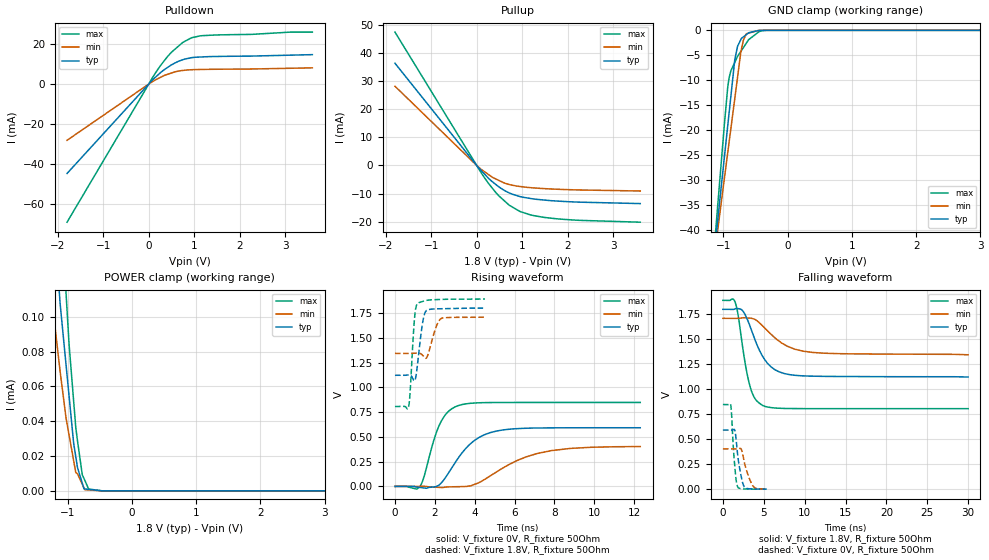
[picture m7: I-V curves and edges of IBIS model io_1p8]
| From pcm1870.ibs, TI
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|   io_1p8 Model
[Model]   io_1p8
Model_type   I/O
Polarity   Non-Inverting
Enable   Active-Low
Vinl = 0.54
Vinh = 1.26
Vmeas = 0.9
Vref = 0.9
Cref = 400pF
Rref = 50
|   typ   min   max
C_comp   2.080e-12   1.781e-12   2.321e-12
[Model spec]
Vinl   0.54   0.513   0.567
Vinh   1.26   1.197   1.323
| Where nom  PVT is Nominal Process, 1.8V, 26C
|   Fast PVT is Strong Process,  1.89V, -40C
|   Slow PVT is Weak Process,   1.71V, 86C
[Voltage Range]   1.8   1.71   1.89
|Ambient Temperature   25   85   -40
|Junction Temperature
[Temperature Range]   26   86   -40
[Pullup Reference]   1.8   1.71   1.89
[Pulldown Reference]   0   0   0
[Power Clamp Reference]   1.8   1.71   1.89
[GND Clamp Reference]   0   0   0
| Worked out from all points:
|   slope of the pulldown table from 0 to 0.27 V, typ, clamps not added: 45.5 ohm
|   slope of the pullup table from 0 to 0.27 V, typ, clamps not added: 57 ohm
|   GND clamp passes 1 mA (typ) near -0.66 V on its own axis
|   falling waveform, V_fixture 1.8V, R_fixture 50Ohm: 20-80 % time 2.31ns typ, 3.44ns min, 1.35ns max; typ from 1.8 V to 1.12 V
|   rising waveform, V_fixture 0V, R_fixture 50Ohm: 20-80 % time 1.43ns typ, 2.4ns min, 824ps max; typ from 0 V to 0.592 V
|   rising waveform, V_fixture 1.8V, R_fixture 50Ohm: 20-80 % time 253ps typ, 336ps min, 190ps max; typ from 1.12 V to 1.8 V
|   falling waveform, V_fixture 0V, R_fixture 50Ohm: 20-80 % time 615ps typ, 872ps min, 408ps max; typ from 0.592 V to 0.001 V
[Pulldown]
|   Voltage   I(typ)   I(min)   I(max)
-1.8V     -44.87mA   -28.23mA   -69.29mA
21.6mV    581uA      343.8uA    910.7uA
178.8mV   4.089mA    2.437mA    6.681mA
333mV     7.078mA    4.214mA    11.46mA
486.9mV   9.444mA    5.428mA    15.66mA
747.7mV   12.18mA    6.802mA    20.86mA
948.1mV   13.24mA    7.173mA    23.24mA
1.177V    13.59mA    7.312mA    24.25mA
2.254V    14mA       7.529mA    24.88mA
3.127V    14.48mA    7.903mA    26.04mA
3.6V      14.73mA    8.105mA    26.04mA
[GND Clamp]
|   Voltage   I(typ)   I(min)   I(max)
-1.8V     -127.5mA   -112.9mA   -149.8mA
-1.095V   -38.91mA   -40.76mA   -36.05mA
-1.053V   -33.64mA   -36.46mA   -29.45mA
-987.3mV  -25.68mA   -29.91mA   -19.15mA
-934.4mV  -19.28mA   -24.66mA   -11.54mA
-909.8mV  -16.3mA    -22.23mA   -9.421mA
-826.2mV  -6.18mA    -13.94mA   -6.495mA
-781.2mV  -3.227mA   -9.481mA   -5.246mA
-727.8mV  -1.815mA   -4.252mA   -4.205mA
-642.3mV  -852.2uA   -679uA     -2.537mA
-348.5mV  -1.381uA   0A         -19.61uA
3.6V      0A         0A         0A
[Pullup]
|   Voltage   I(typ)   I(min)   I(max)
-1.8V     36.4mA     28.23mA    47.51mA
630uV     -48.19uA   -32.61uA   -67.08uA
103.2mV   -1.872mA   -1.451mA   -2.731mA
257.4mV   -4.547mA   -3.209mA   -6.348mA
409.4mV   -6.639mA   -4.724mA   -9.437mA
563.4mV   -8.454mA   -5.933mA   -11.94mA
715.6mV   -9.781mA   -6.799mA   -14.16mA
953.7mV   -11.08mA   -7.49mA    -16.4mA
1.177V    -11.74mA   -7.897mA   -17.59mA
1.481V    -12.32mA   -8.247mA   -18.5mA
2.251V    -13.07mA   -8.732mA   -19.55mA
3.6V      -13.58mA   -9.102mA   -20.21mA
[POWER Clamp]
|   Voltage   I(typ)   I(min)   I(max)
-1.8V     770.7uA    464.9uA    734.5uA
-1.339V   212.5uA    146.7uA    327.1uA
-1.219V   159.1uA    101.4uA    241.9uA
-1.131V   114.8uA    73.11uA    180uA
-1.024V   72.07uA    41.62uA    113uA
-976mV    53.91uA    31.78uA    83.45uA
-873.2mV  19.67uA    10.58uA    36.41uA
-771.8mV  4.398uA    3.838uA    9.223uA
-733mV    1.133uA    714.7nA    6.118uA
-673.6mV  894.9nA    565.2nA    1.093uA
-450mV    0A         0A         0A
3.6V      0A         0A         0A
[Ramp]
R_load = 50
|   typ   min   max
dV/dt_r   0.355124/1.43284e-09   0.241994/2.40645e-09   0.508284/8.22289e-10
dV/dt_f   0.406423/2.31189e-09   0.218829/3.44346e-09   0.650403/1.34999e-09
[Falling Waveform]
V_fixture = 1.8V
V_fixture_min = 1.71V
V_fixture_max = 1.89V
R_fixture = 50Ohm
|   Time   V(typ)   V(min)   V(max)
0s        1.8V       1.71V      1.89V
1.456ns   1.804V     1.71V      1.88V
1.836ns   1.808V     1.71V      1.756V
2.398ns   1.788V     1.715V     1.434V
3.369ns   1.62V      1.712V     1.015V
4.015ns   1.477V     1.695V     896.1mV
4.887ns   1.327V     1.632V     837.5mV
6.91ns    1.173V     1.48V      810.3mV
9.834ns   1.134V     1.381V     806.6mV
30ns      1.123V     1.345V     806mV
[Rising Waveform]
V_fixture = 0V
V_fixture_min = 0V
V_fixture_max = 0V
R_fixture = 50Ohm
|   Time   V(typ)   V(min)   V(max)
0s        333pV      635.1pV    252.7pV
1.239ns   -10.3mV    545.1uV    -5.089mV
1.456ns   -15.7mV    1.567mV    96.74mV
2.27ns    24.25mV    -10.17mV   636.9mV
2.709ns   142.7mV    -4.597mV   761.4mV
3.182ns   288.2mV    -2.652mV   815.7mV
4.195ns   491.3mV    35.93mV    843.5mV
5.473ns   571.4mV    192.4mV    846.7mV
7.864ns   590.7mV    361.7mV    847.1mV
12.31ns   591.8mV    402.3mV    847.1mV
[Rising Waveform]
V_fixture = 1.8V
V_fixture_min = 1.71V
V_fixture_max = 1.89V
R_fixture = 50Ohm
|   Time   V(typ)   V(min)   V(max)
0s        1.121V     1.342V     806mV
681.7ps   1.125V     1.342V     800.7mV
764ps     1.123V     1.342V     961.4mV
966.4ps   1.068V     1.343V     1.658V
1.12ns    1.212V     1.345V     1.842V
1.38ns    1.642V     1.324V     1.865V
1.574ns   1.774V     1.295V     1.877V
2.109ns   1.791V     1.631V     1.885V
2.332ns   1.792V     1.695V     1.886V
4.515ns   1.799V     1.707V     1.89V
[Falling Waveform]
V_fixture = 0V
V_fixture_min = 0V
V_fixture_max = 0V
R_fixture = 50Ohm
|   Time   V(typ)   V(min)   V(max)
0s        591.9mV    403.3mV    847.1mV
966.4ps   591.5mV    403.1mV    842mV
1.454ns   590.7mV    402.9mV    231.4mV
1.626ns   492.6mV    402.9mV    89.47mV
1.807ns   344.8mV    404.4mV    23.62mV
2.264ns   119.1mV    397.6mV    4.52mV
2.615ns   23.11mV    274.3mV    2.531mV
3.182ns   4.607mV    119.3mV    1.467mV
3.813ns   2.023mV    19.36mV    710.7uV
5.359ns   654.3uV    1.448mV    348.4uV
